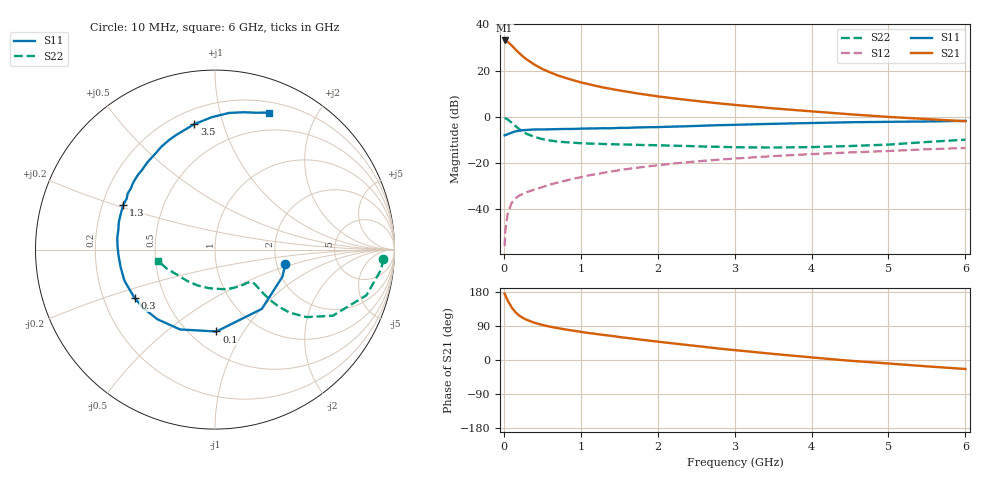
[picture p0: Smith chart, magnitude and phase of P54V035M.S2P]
! SIEMENS Small Signal Semiconductors
! BFP183
! Si NPN RF Bipolar Junction Transistor in SOT143
! VCE = 4 V  IC = 35 mA
! Common Emitter S-Parameters:  March  1996
# GHz  S  MA  R  50
!  f  S11  S21  S12  S22
! GHz  MAG  ANG  MAG  ANG  MAG  ANG  MAG  ANG
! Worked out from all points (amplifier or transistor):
!   36 points, 10 MHz to 6 GHz, reference 50 ohm
!   highest |S21| = 33.1 dB at 10 MHz (marker M1)
!   |S21| within 3 dB of that: start of sweep to 125.4 MHz
!   unconditionally stable (mu >= 1): 585.6 MHz to 5.693 GHz
!   at 250 MHz: K = 0.64, MSG = 29.7 dB, |S12| = -33.4 dB
!   at 1.4 GHz: K = 1.19, MAG = 15.2 dB, |S12| = -23.6 dB
!   at 6 GHz: K = 0.96, MSG = 5.8 dB, |S12| = -13.5 dB
!   S11 on the Smith chart (normalised r, x): 10 MHz: 2.24, -0.41; 100 MHz: 0.66, -0.77; 300 MHz: 0.33, -0.25; 1.3 GHz: 0.29, +0.21; 3.5 GHz: 0.29, +0.81; 6 GHz: 0.31, +1.42
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0.01  0.4001 -11.2  44.97 175.1  0.0016 83.2  0.9394 -3.1
0.02  0.4051 -21.9  44.83 170.6  0.0035 81.8  0.9325 -6.8
0.05  0.4209 -51.7  42.22 157.0  0.008 76.8  0.881 -16.8
0.1  0.4563 -89.0  35.19 139.2  0.0137 60.5  0.7528 -29.3
0.15  0.4856 -113.6  28.9 126.3  0.0171 56.2  0.6339 -36.4
0.2  0.5035 -129.6  23.92 117.3  0.02 53.8  0.5436 -40.2
0.25  0.5147 -140.3  20.15 110.7  0.0215 51.3  0.4769 -41.8
0.3  0.5231 -149.0  17.37 105.9  0.0236 52.3  0.4283 -42.3
0.4  0.5335 -161.0  13.46 98.1  0.0269 53.4  0.3679 -42.3
0.5  0.5349 -169.6  10.88 92.5  0.0303 54.3  0.3314 -41.7
0.6  0.5385 -176.6  9.223 88.0  0.0343 55.8  0.3082 -41.2
0.7  0.5439 177.7  7.893 84.1  0.0381 57.0  0.2936 -41.0
0.8  0.5486 172.9  6.984 80.6  0.0416 57.6  0.2836 -41.1
1.1  0.5606 160.3  5.103 71.3  0.0542 58.5  0.2651 -43.0
1.3  0.5688 153.9  4.3 66.0  0.062 57.7  0.2592 -45.5
1.7  0.5882 141.1  3.289 55.7  0.0784 55.5  0.2503 -52.1
2.2  0.6158 127.5  2.526 43.8  0.0977 51.5  0.238 -62.4
2.8  0.6612 113.0  1.958 30.1  0.119 45.7  0.2255 -78.0
3.5  0.7084 99.4  1.531 16.1  0.1418 39.4  0.2176 -99.3
4.5  0.7656 84.1  1.139 -2.0  0.1701 29.8  0.2344 -132.4
5.5  0.7958 73.4  0.897 -16.8  0.1996 21.6  0.2869 -157.7
6  0.8199 68.6  0.805 -23.7  0.2124 17.0  0.3215 -168.4
